FUNCTION_BLOCK FB_LN_IED_LD1_LEDGGIO2 EXTENDS FB_AcsiCommonLogicalNodeClass
VAR_INPUT
	NamPlt: FB_DO_IED_LD1_LEDGGIO2_NamPlt := (sClass:='LPL', bLinkResult:=THIS^.AddDataToContainer(ipData:=NamPlt));
	Beh: FB_DO_IED_LD1_LEDGGIO2_Beh := (sClass:='ENS', bLinkResult:=THIS^.AddDataToContainer(ipData:=Beh));
	Health: FB_DO_IED_LD1_LEDGGIO2_Health := (sClass:='ENS', bLinkResult:=THIS^.AddDataToContainer(ipData:=Health));
	Mod_: FB_DO_IED_LD1_LEDGGIO2_Mod := (sObjectName:='Mod', sClass:='ENC', bLinkResult:=THIS^.AddDataToContainer(ipData:=Mod_));
	SPCSO1: FB_DO_IED_LD1_LEDGGIO2_SPCSO1 := (sClass:='SPC', bLinkResult:=THIS^.AddDataToContainer(ipData:=SPCSO1));
END_VAR
VAR
END_VAR

END_FUNCTION_BLOCK
